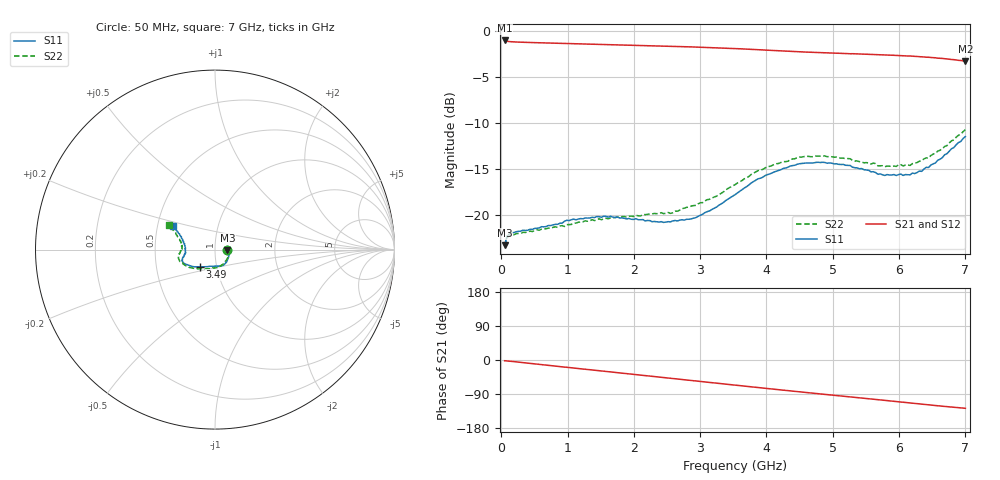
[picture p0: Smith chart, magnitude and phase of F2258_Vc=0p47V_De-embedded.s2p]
! Integrated Device Technology
! Corporate Headquarters
! 6024 Silver Creek Valley Road
! San Jose, CA 95138  USA
! Phone:  1-408-284-8200
! Toll Free:  1-800-223-1366
! Webpage:  http://www.idt.com/
! Timing and RF Division
! 515 Groton Road, Suite 102
! Westford, MA 01886-6024
! Device:  F2258
! Description: Voltage Variable RF Attenuator
! Frequency:  50.0 -  6000.00 MHz
! Package:  3x3 mm Thin QFN Plastic Package: 16 pin
! Ports:  2 RF, 2 DC
!  Pin  1  = NC
!  Pin  2  = NC
!  Pin  3  = RF2  = Port 2
!  Pin  4  = GND
!  Pin  5  = Vdd
!  Pin  6  = NC
!  Pin  7  = VCTRL
!  Pin  8  = NC
!  Pin  9  = GND
!  Pin 10  = RF1  = Port 1
!  Pin 11  = NC
!  Pin 12  = NC
!  Pin 13  = NC
!  Pin 14  = NC
!  Pin 15  = NC
!  Pin 16  = NC
! Vcntrl:  0.470 Volts
! Vdd:  +3.300 Volts
! Current:  1.099 mA
! Data:  The device was measured on a the F2258 evaluation board which has
!  individual transmission lines to the RF pins.  Data was collected
!  using a calibrated network analyzer.  The evaluation board was
!  de-embedded using a TRL calibration technique.
!  The reference plane is the edge of the package pin.
! Misc:  SN 10
!  Action Tracker AT0285
! Date Measured:  2014-12-10
! Date:  2016-01-13  MJV
! Note:
!  Integrated Device Technology supplies this data as a sample of measured
!  data at the package pin for this product.  Your particular data for this
!  product may vary.
!  Data was taken at 25 degrees C.
!  Integrated Device Technology reserves the right to change this data at anytime.
!Freq_(GHz)  S11M_(dB)  S11P_(deg)  S21M_(dB)  S21P_(deg)  S12M_(dB)  S12P_(deg)  S22M_(dB)  S22P_(deg)
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# GHz S dB R 50
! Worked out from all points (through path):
!   201 points, 50 MHz to 7 GHz, reference 50 ohm
!   highest |S21| = -1.07 dB at 50 MHz (marker M1); lowest = -3.3 dB at 7 GHz (marker M2)
!   group delay of S21, straight-line fit = 50.5 ps
!   lowest |S11| = -23.2 dB at 50 MHz (marker M3), VSWR 1.15, Z = 57.4 - j0.437 ohm
!   |S11| at or under -10 dB: start of sweep to end of sweep
!   |S22| runs from -23.4 to -10.7 dB; largest |S21 - S12| = 0.00045
!   S11 on the Smith chart (normalised r, x): 50 MHz: 1.15, -0.01; 3.49 GHz: 0.83, -0.16; 7 GHz: 0.61, +0.17
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0.05  -23.25 -3.2  -1.07 -2.0  -1.07 -2.0  -23.36 -3.1
0.08475  -22.32 -5.2  -1.15 -2.5  -1.15 -2.5  -22.47 -5.0
0.15425  -21.88 -8.0  -1.21 -3.7  -1.21 -3.7  -22.11 -8.8
0.71025  -21.12 -32.9  -1.35 -14.1  -1.35 -14.1  -21.40 -36.0
1.2315  -20.39 -53.6  -1.46 -23.8  -1.46 -23.8  -20.72 -60.1
1.6485  -20.13 -64.7  -1.54 -31.4  -1.54 -31.4  -20.31 -73.2
2.37825  -20.75 -84.6  -1.67 -44.8  -1.67 -44.8  -19.82 -91.5
2.552  -20.74 -90.4  -1.70 -48.0  -1.70 -48.0  -19.81 -96.8
2.93425  -20.27 -107.1  -1.78 -55.1  -1.78 -55.1  -18.94 -110.4
3.247  -19.12 -120.5  -1.86 -61.0  -1.86 -61.0  -17.95 -122.7
3.49025  -17.93 -130.8  -1.94 -65.6  -1.94 -65.6  -16.83 -132.0
3.525  -17.78 -131.8  -1.95 -66.2  -1.95 -66.2  -16.70 -133.5
4.0115  -15.61 -146.8  -2.13 -75.3  -2.13 -75.2  -14.76 -149.3
4.46325  -14.48 -155.9  -2.29 -83.4  -2.29 -83.4  -13.76 -160.7
4.7065  -14.34 -159.2  -2.36 -87.7  -2.36 -87.7  -13.66 -165.0
5.2625  -14.62 -165.9  -2.51 -97.4  -2.51 -97.4  -13.89 -173.3
5.6795  -15.57 -172.3  -2.60 -104.6  -2.60 -104.6  -14.66 -178.9
5.85325  -15.66 -176.5  -2.65 -107.8  -2.65 -107.8  -14.69 176.5
6.166  -15.63 175.5  -2.76 -113.4  -2.76 -113.3  -14.61 170.4
6.33975  -15.25 168.9  -2.84 -116.5  -2.84 -116.5  -14.10 165.9
6.722  -13.34 156.3  -3.07 -123.1  -3.07 -123.1  -12.47 156.8
7  -11.48 150.3  -3.31 -127.4  -3.32 -127.4  -10.74 151.8
